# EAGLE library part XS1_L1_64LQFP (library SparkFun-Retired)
XMos processor (multicore) Not in catalog
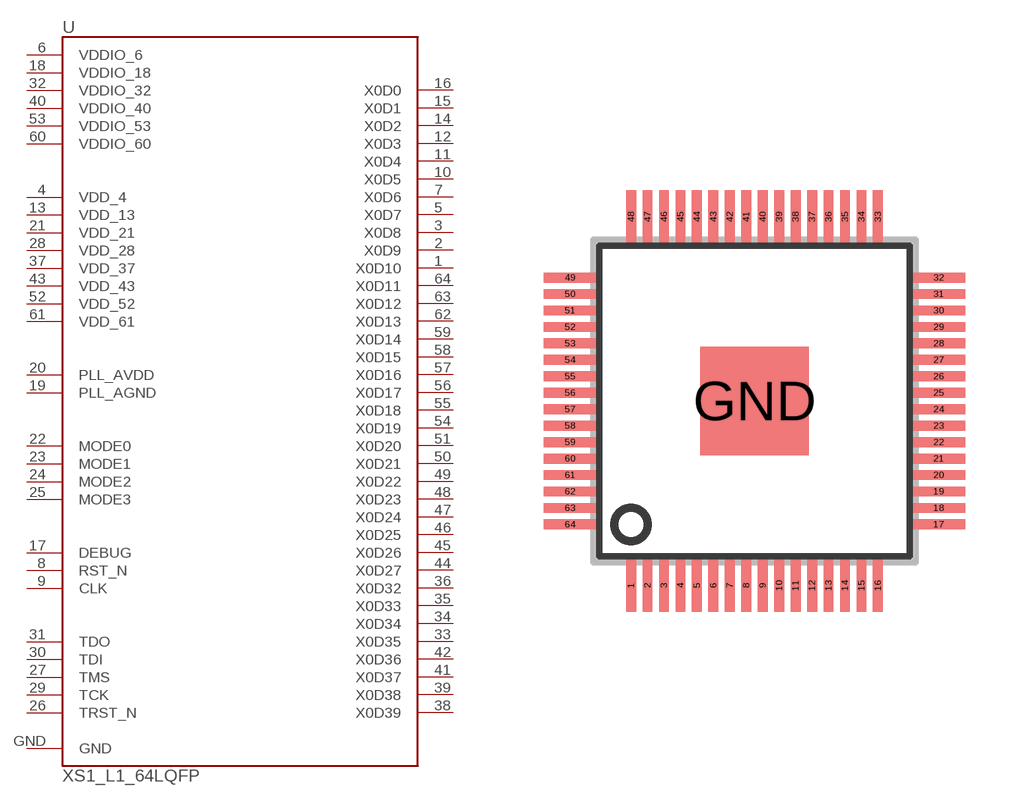
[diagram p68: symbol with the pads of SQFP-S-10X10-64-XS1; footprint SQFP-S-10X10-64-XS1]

Designator prefix -

## XS1_L1_64LQFP  [SQFP-S-10X10-64-XS1]
1  X0D10
2  X0D9
3  X0D8
4  VDD_4
5  X0D7
6  VDDIO_6
7  X0D6
8  RST_N
9  CLK
10  X0D5
11  X0D4
12  X0D3
13  VDD_13
14  X0D2
15  X0D1
16  X0D0
17  DEBUG
18  VDDIO_18
19  PLL_AGND
20  PLL_AVDD
21  VDD_21
22  MODE0
23  MODE1
24  MODE2
25  MODE3
26  TRST_N
27  TMS
28  VDD_28
29  TCK
30  TDI
31  TDO
32  VDDIO_32
33  X0D35
34  X0D34
35  X0D33
36  X0D32
37  VDD_37
38  X0D39
39  X0D38
40  VDDIO_40
41  X0D37
42  X0D36
43  VDD_43
44  X0D27
45  X0D26
46  X0D25
47  X0D24
48  X0D23
49  X0D22
50  X0D21
51  X0D20
52  VDD_52
53  VDDIO_53
54  X0D19
55  X0D18
56  X0D17
57  X0D16
58  X0D15
59  X0D14
60  VDDIO_60
61  VDD_61
62  X0D13
63  X0D12
64  X0D11
GND  GND

## Footprint SQFP-S-10X10-64-XS1 (pad centres in mm)
smd 0.3 x 1.6: 1 -3.75,-5.6; 2 -3.25,-5.6; 3 -2.75,-5.6; 4 -2.25,-5.6; 5 -1.75,-5.6; 6 -1.25,-5.6; 7 -0.75,-5.6; 8 -0.25,-5.6; 9 0.25,-5.6; 10 0.75,-5.6; 11 1.25,-5.6; 12 1.75,-5.6; 13 2.25,-5.6; 14 2.75,-5.6; 15 3.25,-5.6; 16 3.75,-5.6; 33 3.75,5.6; 34 3.25,5.6; 35 2.75,5.6; 36 2.25,5.6; 37 1.75,5.6; 38 1.25,5.6; 39 0.75,5.6; 40 0.25,5.6; 41 -0.25,5.6; 42 -0.75,5.6; 43 -1.25,5.6; 44 -1.75,5.6; 45 -2.25,5.6; 46 -2.75,5.6; 47 -3.25,5.6; 48 -3.75,5.6
smd 1.6 x 0.3: 17 5.6,-3.75; 18 5.6,-3.25; 19 5.6,-2.75; 20 5.6,-2.25; 21 5.6,-1.75; 22 5.6,-1.25; 23 5.6,-0.75; 24 5.6,-0.25; 25 5.6,0.25; 26 5.6,0.75; 27 5.6,1.25; 28 5.6,1.75; 29 5.6,2.25; 30 5.6,2.75; 31 5.6,3.25; 32 5.6,3.75; 49 -5.6,3.75; 50 -5.6,3.25; 51 -5.6,2.75; 52 -5.6,2.25; 53 -5.6,1.75; 54 -5.6,1.25; 55 -5.6,0.75; 56 -5.6,0.25; 57 -5.6,-0.25; 58 -5.6,-0.75; 59 -5.6,-1.25; 60 -5.6,-1.75; 61 -5.6,-2.25; 62 -5.6,-2.75; 63 -5.6,-3.25; 64 -5.6,-3.75
smd 3.3 x 3.3: GND 0,0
